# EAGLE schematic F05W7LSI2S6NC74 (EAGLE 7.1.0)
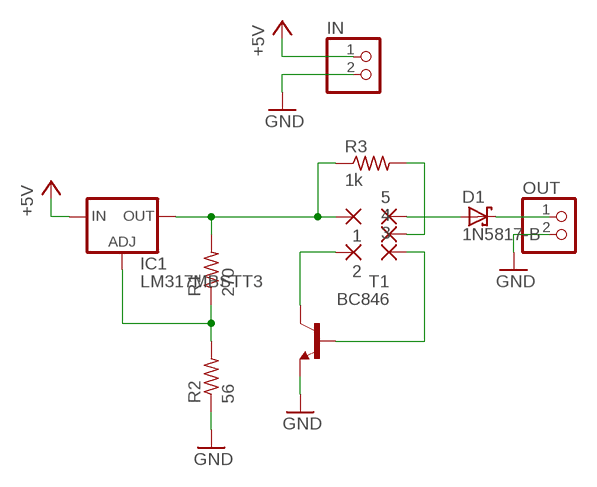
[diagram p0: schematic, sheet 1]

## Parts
1  SMD2  [SMD1,27-2,54]
2  SMD2  [SMD1,27-2,54]
3  SMD2  [SMD1,27-2,54]
4  SMD2  [SMD1,27-2,54]
5  SMD2  [SMD1,27-2,54]
D1  1N5817-B  [DO41-7.6]
IC1  LM317MBSTT3  [SOT223]
IN  PINHD-1X2  [1X02]
OUT  PINHD-1X2  [1X02]
R1  270  R-US_R0805  [R0805]
R2  56  R-US_R0805  [R0805]
R3  1k  R-US_R0805  [R0805]
T1  BC846  [SOT23]

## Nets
+5V: IC1.3(IN) IN.1
GND: IN.2 OUT.2 R2.1 T1.2(E)
N$1: 1.1(P) IC1.4(OUT) R1.2 R3.1
N$2: IC1.1(ADJ) R1.1 R2.2
N$3: 5.1(P) D1.A
N$4: 3.1(P) T1.1(B)
N$5: 2.1(P) T1.3(C)
N$6: 4.1(P) R3.2
N$7: D1.C OUT.1

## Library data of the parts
1-5 = wirepad:SMD2: SMD PAD
D1 = diode:1N581*: 1.0A SCHOTTKY BARRIER RECTIFIER
IC1 = v-reg:LM317?*: 500 mA Adjustable Output Positive Voltage Regulator Source: http://www.onsemi.co.jp .. LM317M-D.PDF
IN OUT = pinhead:PINHD-1X2: PIN HEADER
R1-R3 = rcl:R-US_: RESISTOR, American symbol
T1 = transistor:BC846: NPN TRANSISTOR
